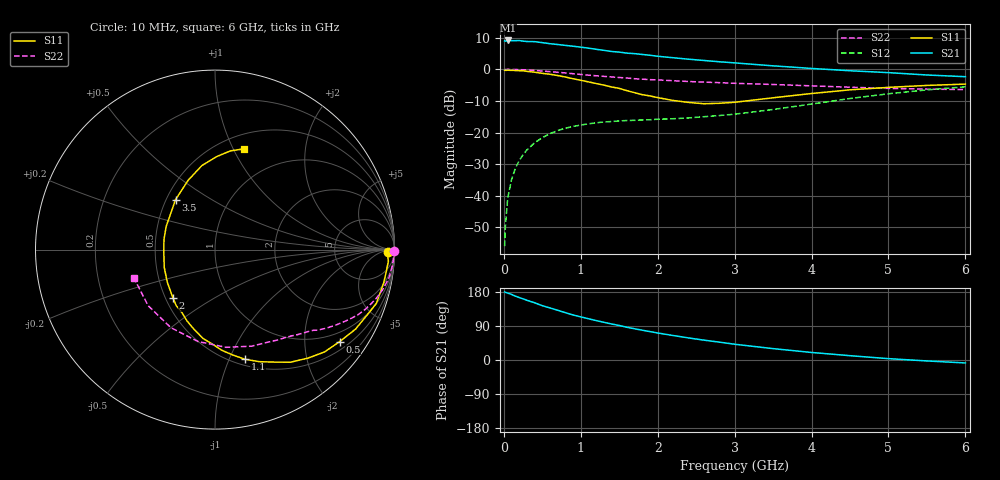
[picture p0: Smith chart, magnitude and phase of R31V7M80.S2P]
! SIEMENS Small Signal Semiconductors
! BFR181
! Si NPN RF Bipolar Junction Transistor in SOT23
! VCE = 1.75 V  IC = 0.8 mA
! Common Emitter S-Parameters:  May  1996
# GHz  S  MA  R  50
!  f  S11  S21  S12  S22
! GHz  MAG  ANG  MAG  ANG  MAG  ANG  MAG  ANG
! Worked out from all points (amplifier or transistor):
!   36 points, 10 MHz to 6 GHz, reference 50 ohm
!   highest |S21| = 9.1 dB at 50 MHz (marker M1)
!   |S21| within 3 dB of that: start of sweep to 1.263 GHz
!   unconditionally stable (mu >= 1): 2.101 GHz to 3.808 GHz
!   at 250 MHz: K = 0.15, MSG = 18.0 dB, |S12| = -27.0 dB
!   at 1.4 GHz: K = 0.72, MSG = 11.1 dB, |S12| = -16.5 dB
!   at 6 GHz: K = 0.90, MSG = 1.6 dB, |S12| = -5.5 dB
!   S11 on the Smith chart (normalised r, x): 10 MHz: 52, -19; 500 MHz: 0.72, -2.88; 1.1 GHz: 0.56, -1.14; 2 GHz: 0.55, -0.34; 3.5 GHz: 0.56, +0.36; 6 GHz: 0.65, +1.10
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0.01  0.9666 -0.7  2.811 179.6  0.0016 90.2  1 -0.4
0.02  0.9606 -1.4  2.78 178.5  0.0033 83.5  0.9902 -0.7
0.05  0.9682 -3.8  2.858 176.5  0.0091 86.4  0.9981 -1.8
0.1  0.9619 -7.4  2.839 173.1  0.0181 85.9  0.9948 -3.5
0.15  0.9581 -11.1  2.837 168.4  0.0272 82.4  0.9922 -5.3
0.2  0.951 -14.8  2.848 164.9  0.0361 79.9  0.9872 -7.0
0.3  0.9277 -22.2  2.751 157.6  0.0532 75.6  0.9764 -10.3
0.4  0.8997 -29.5  2.736 151.0  0.0689 70.8  0.9597 -13.6
0.5  0.8634 -36.4  2.64 143.3  0.083 66.5  0.9396 -16.7
0.8  0.7552 -56.2  2.388 124.9  0.1172 55.3  0.876 -24.4
0.9  0.7093 -62.1  2.318 118.8  0.125 52.4  0.8522 -26.6
1.1  0.6328 -74.8  2.161 108.9  0.1376 47.6  0.8091 -30.5
1.3  0.5623 -86.1  1.995 99.5  0.147 43.7  0.7733 -33.8
1.6  0.4594 -104.7  1.801 86.4  0.1551 40.2  0.7291 -38.0
2  0.3571 -131.0  1.608 71.3  0.1624 39.9  0.6796 -43.0
2.2  0.3219 -145.7  1.524 64.6  0.1654 40.3  0.6599 -45.9
2.6  0.2856 -177.5  1.379 52.4  0.178 43.3  0.6271 -51.4
3  0.3011 154.6  1.264 41.6  0.1952 46.6  0.6008 -58.2
3.5  0.3546 128.3  1.135 30.0  0.2317 49.3  0.5752 -69.3
4.5  0.4738 98.9  0.949 11.4  0.3453 46.6  0.5206 -100.6
5.5  0.5563 81.2  0.813 -2.5  0.4729 34.1  0.4862 -140.0
6  0.5834 74.2  0.764 -7.8  0.529 25.9  0.4783 -160.4
